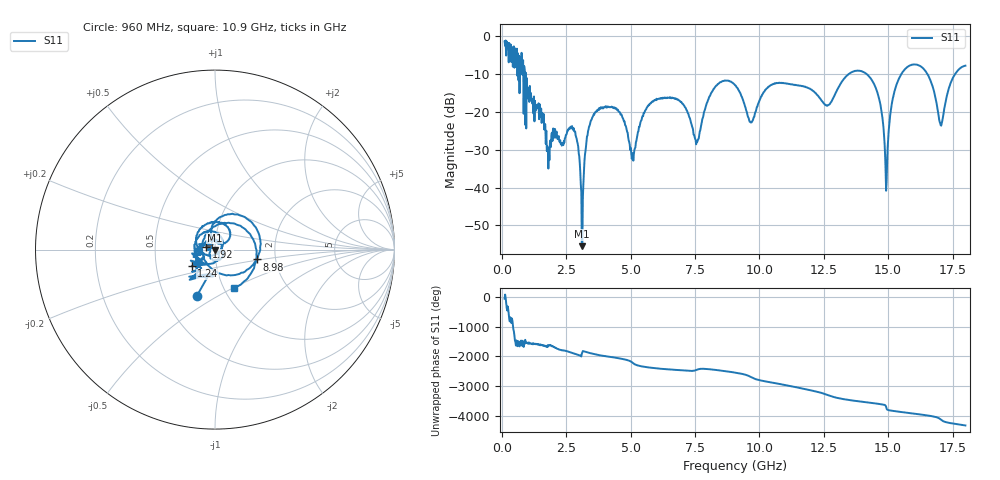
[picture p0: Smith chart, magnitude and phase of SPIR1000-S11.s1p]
!Keysight Technologies,P9374A,MY57211922,A.15.40.13
!Date: Friday, December 22, 2023 10:05:48
!Correction: S11(C  1-Port  )
!S1P File: Measurement: S11:
# Hz S  dB  R 50
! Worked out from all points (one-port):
!   896 points, 100 MHz to 18 GHz, reference 50 ohm
!   lowest |S11| = -55.5 dB at 3.1 GHz (marker M1), VSWR 1.00, Z = 49.9 - j0.159 ohm
!   |S11| at or under -10 dB: 920.5 MHz to 13.47 GHz (12.55 GHz wide, 174 % of centre); 14.16 GHz to 15.51 GHz (1.349 GHz wide, 9.09 % of centre); 16.53 GHz to 17.6 GHz (1.075 GHz wide, 6.3 % of centre)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
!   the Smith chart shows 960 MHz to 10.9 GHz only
!   S11 on the Smith chart (normalised r, x): 960 MHz: 0.72, -0.41; 1.24 GHz: 0.76, -0.14; 1.92 GHz: 0.91, +0.03; 8.98 GHz: 1.59, -0.19; 10.9 GHz: 1.12, -0.51
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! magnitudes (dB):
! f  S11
! 100 MHz  -1.4
! 960 MHz  -11.1
! 1.24 GHz  -15.9
! 1.92 GHz  -25.8
! 2.34 GHz  -28.6
! 2.8 GHz  -25.1
! 3.1 GHz  -55.5
! 3.52 GHz  -21.3
! 4.58 GHz  -20.1
! 5.1 GHz  -32.9
! 5.7 GHz  -18.1
! 6.82 GHz  -16.8
! 7.56 GHz  -27.9
! 8.2 GHz  -14.2
! 8.98 GHz  -12.5
! 9.06 GHz  -13.0
! 9.68 GHz  -22.8
! 10.9 GHz  -12.4
! 11.3 GHz  -12.8
! 12.64 GHz  -18.4
! 13.54 GHz  -9.7
! 14.5 GHz  -13.4
! 14.92 GHz  -40.8
! 15.22 GHz  -15.3
! 15.78 GHz  -8.0
! 16.52 GHz  -9.9
! 17.04 GHz  -23.5
! 18 GHz  -7.8
